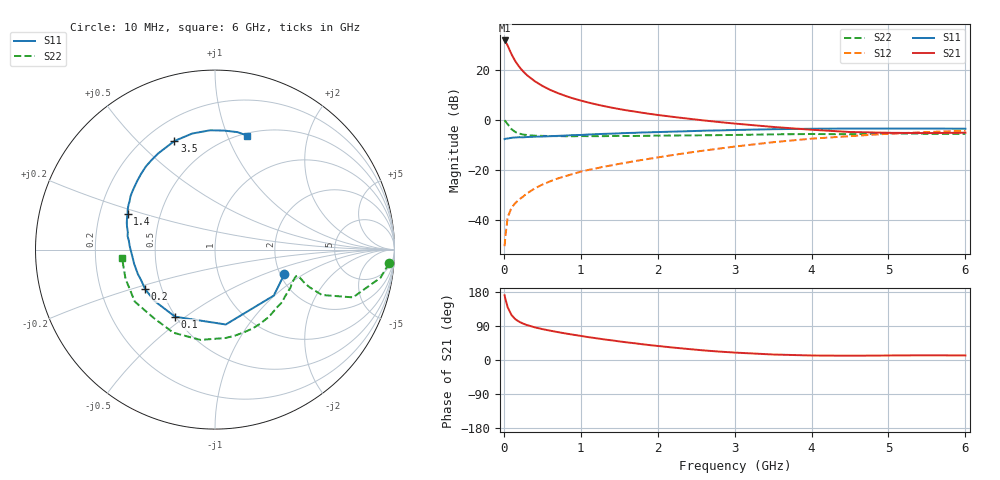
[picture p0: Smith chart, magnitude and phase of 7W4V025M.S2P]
! Infineon Technologies  Discrete & RF Semiconductors
! BFS17W
! Si NPN RF Bipolar Junction Transistor in SOT323
! VCE = 4 V  IC = 25 mA
! Common Emitter S-Parameters:  August  1999
# GHz  S  MA  R  50
!  f  S11  S21  S12  S22
! GHz  MAG  ANG  MAG  ANG  MAG  ANG  MAG  ANG
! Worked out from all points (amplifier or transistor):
!   36 points, 10 MHz to 6 GHz, reference 50 ohm
!   highest |S21| = 31.6 dB at 10 MHz (marker M1)
!   |S21| within 3 dB of that: start of sweep to 63.25 MHz
!   unconditionally stable (mu >= 1): 235.1 MHz to 2.184 GHz; 4.962 GHz to end of sweep
!   at 250 MHz: K = 1.04, MAG = 23.8 dB, |S12| = -30.7 dB
!   at 1.4 GHz: K = 1.17, MAG = 9.0 dB, |S12| = -18.2 dB
!   at 6 GHz: K = 1.06, MAG = -1.9 dB, |S12| = -4.4 dB
!   S11 on the Smith chart (normalised r, x): 10 MHz: 2.10, -0.69; 100 MHz: 0.50, -0.46; 200 MHz: 0.40, -0.22; 1.4 GHz: 0.32, +0.18; 3.5 GHz: 0.31, +0.65; 6 GHz: 0.53, +1.18
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0.01  0.4098 -19.6  38.05 170.7  0.003 82.9  0.9731 -4.5
0.02  0.4159 -38.0  36.85 161.2  0.0047 83.2  0.9358 -9.6
0.05  0.4215 -81.8  29.91 139.1  0.0113 67.9  0.8136 -19.1
0.1  0.435 -120.7  20.15 118.5  0.0176 59.6  0.6472 -23.0
0.15  0.4422 -139.6  14.6 107.5  0.0218 60.5  0.5664 -21.7
0.2  0.4472 -150.3  11.35 100.9  0.0258 62.7  0.5284 -20.2
0.25  0.4456 -157.7  9.221 96.0  0.0292 63.9  0.506 -18.8
0.3  0.4509 -162.5  7.755 92.3  0.0339 65.9  0.4947 -18.2
0.4  0.4575 -170.1  5.882 86.3  0.0423 68.1  0.48 -17.8
0.5  0.4617 -175.0  4.727 81.6  0.0507 69.4  0.4756 -18.2
0.6  0.4684 -179.0  3.945 77.5  0.0588 70.8  0.472 -19.3
0.7  0.4753 177.8  3.402 73.7  0.0672 71.0  0.4699 -20.8
0.9  0.4924 171.3  2.661 66.8  0.0829 71.8  0.4678 -24.5
1.1  0.5065 165.4  2.194 60.3  0.0994 72.4  0.4693 -28.9
1.4  0.5262 157.7  1.741 51.9  0.1226 72.9  0.4727 -36.4
1.8  0.556 148.0  1.374 41.6  0.1576 73.4  0.4752 -47.5
2.2  0.5775 138.8  1.138 32.8  0.1976 72.9  0.4837 -58.9
2.8  0.6116 125.2  0.897 22.2  0.2655 69.9  0.492 -77.1
3.5  0.646 110.5  0.717 14.5  0.3555 63.5  0.5095 -99.1
4.5  0.6654 92.3  0.568 11.3  0.4693 50.3  0.512 -132.5
5.5  0.6663 79.1  0.54 12.4  0.5663 37.3  0.5244 -161.9
6  0.6598 74.1  0.55 12.0  0.6042 31.0  0.5201 -174.9
